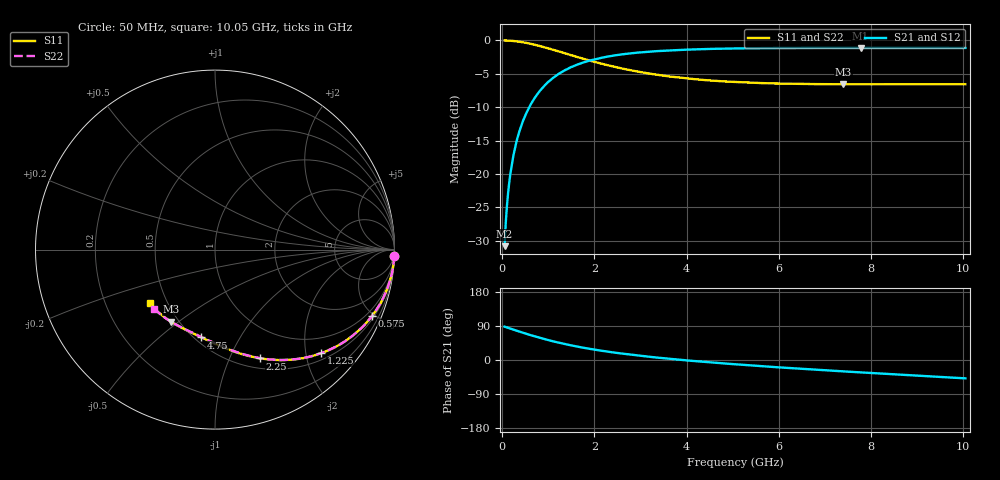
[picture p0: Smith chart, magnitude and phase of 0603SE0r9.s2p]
! AVX Thin Film Operation		Date: August 2001
! Description: Accu-P® Series, Thin Film, SMD, RF Capacitor
! Part Number: 06035J0R9ABT
! 50 MHz  -  10.05 GHz
! Serial Measurements
# mhz S db R 50
!	S11		S21		S12		S22
!	dB	Phase	dB	Phase	dB	Phase	dB	Phase
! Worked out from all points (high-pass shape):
!   401 points, 50 MHz to 10.05 GHz, reference 50 ohm
!   highest |S21| = -1.11 dB at 7.775 GHz (marker M1); lowest = -30.8 dB at 50 MHz (marker M2)
!   |S21| within 3 dB of the highest: 1.46 GHz to end of sweep
!   lowest |S11| = -6.6 dB at 7.4 GHz (marker M3), VSWR 2.77, Z = 22.8 - j23.5 ohm
!   |S11| at or under -10 dB: nowhere
!   |S22| runs from -6.5 to 0.0 dB; largest |S21 - S12| = 0
!   S11 on the Smith chart (normalised r, x): 50 MHz: 1, -56; 575 MHz: 0.64, -4.87; 1.225 GHz: 0.63, -2.31; 2.25 GHz: 0.61, -1.31; 4.75 GHz: 0.54, -0.70; 10.05 GHz: 0.40, -0.30
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50  -0.00 -2.1  -30.80 87.9  -30.80 87.9  -0.00 -2.1
75  -0.01 -3.1  -27.31 87.0  -27.31 87.0  -0.01 -3.1
125  -0.02 -5.1  -22.89 84.9  -22.89 84.9  -0.02 -5.1
150  -0.03 -6.1  -21.31 83.9  -21.31 83.9  -0.03 -6.1
200  -0.06 -8.2  -18.88 81.8  -18.88 81.8  -0.06 -8.2
250  -0.09 -10.2  -16.94 79.8  -16.94 79.8  -0.09 -10.2
325  -0.15 -13.2  -14.69 76.8  -14.69 76.8  -0.15 -13.2
400  -0.22 -16.2  -13.03 73.8  -13.03 73.8  -0.22 -16.2
575  -0.45 -22.8  -10.14 67.1  -10.14 67.1  -0.45 -22.8
850  -0.90 -32.6  -7.27 57.4  -7.27 57.4  -0.90 -32.6
1225  -1.65 -44.2  -5.00 45.7  -5.00 45.7  -1.65 -44.2
1725  -2.68 -56.8  -3.38 33.2  -3.38 33.2  -2.68 -56.8
2250  -3.65 -67.4  -2.46 22.7  -2.46 22.7  -3.65 -67.2
2800  -4.48 -76.2  -1.92 13.8  -1.92 13.8  -4.48 -75.9
3400  -5.18 -84.3  -1.58 5.9  -1.58 5.9  -5.17 -83.8
4750  -6.11 -98.9  -1.24 -8.5  -1.24 -8.5  -6.09 -97.8
5050  -6.22 -101.6  -1.20 -11.3  -1.20 -11.3  -6.21 -100.6
6725  -6.53 -115.9  -1.11 -25.1  -1.11 -25.1  -6.51 -113.9
7400  -6.56 -121.3  -1.11 -30.0  -1.11 -30.0  -6.54 -118.3
7775  -6.56 -124.0  -1.11 -32.8  -1.11 -32.8  -6.54 -121.0
8400  -6.56 -129.2  -1.11 -37.2  -1.11 -37.2  -6.53 -125.2
10050  -6.55 -140.8  -1.12 -48.4  -1.12 -48.4  -6.52 -135.8
